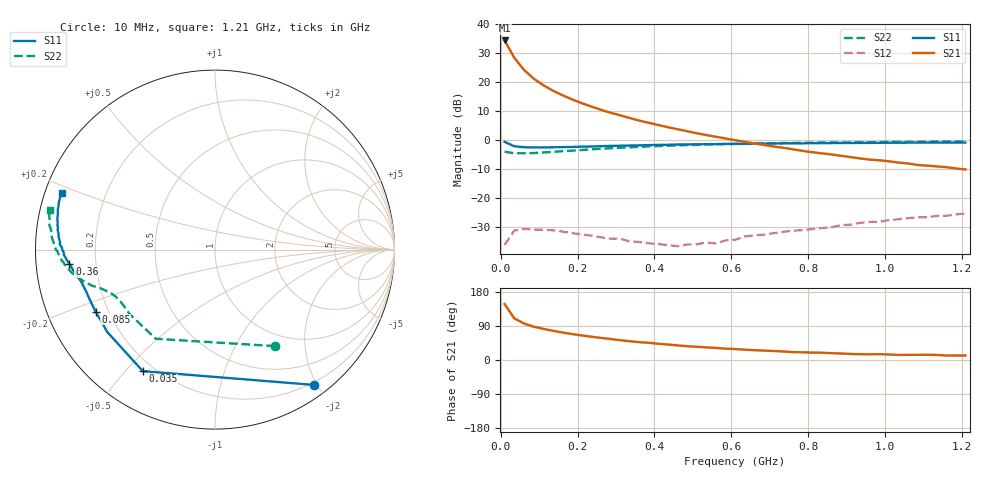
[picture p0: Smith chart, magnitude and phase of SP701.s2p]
!  POLYFET RF DEVICES
!  S PARAMETERS FOR
!  SP701
!  VDS=28, IDQ=200MA
! S1A1Die, AP pkg, Vds=28Vdc, Idq=200ma, Vgsth=2.60Vdc
! Date: Thu Jul 23 11:46:25 1998
# MHZ  S  MA  R  50.0000
! SCATTERING PARAMETERS :
! Freq=MHz Mag[s11] Ang[s11] Mag[s21] Ang[s21] Mag[s12] Ang[s12] Mag[s22] Ang[s22]
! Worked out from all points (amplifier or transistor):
!   49 points, 10 MHz to 1.21 GHz, reference 50 ohm
!   highest |S21| = 34.3 dB at 10 MHz (marker M1)
!   |S21| within 3 dB of that: start of sweep to 22.7 MHz
!   unconditionally stable (mu >= 1): 301.8 MHz to end of sweep
!   at 210 MHz: K = 0.66, MSG = 22.6 dB, |S12| = -32.4 dB
!   at 610 MHz: K = 1.67, MAG = 12.3 dB, |S12| = -34.3 dB
!   at 1.21 GHz: K = 1.05, MAG = 6.2 dB, |S12| = -25.2 dB
!   S11 on the Smith chart (normalised r, x): 10 MHz: 0.17, -1.96; 35 MHz: 0.16, -0.56; 85 MHz: 0.15, -0.24; 360 MHz: 0.10, -0.05; 1.21 GHz: 0.05, +0.18
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10  0.9341 -53.8  52.1 147.7  0.01566 58.0  0.6334 -58.1
35  0.7876 -120.7  26.4 110.0  0.02777 24.4  0.5962 -123.5
60  0.7556 -142.5  16.32 96.4  0.02968 13.1  0.5961 -142.8
85  0.7494 -152.6  11.58 88.1  0.02891 6.8  0.5998 -150.8
110  0.7513 -158.1  8.905 82.3  0.02883 3.8  0.6133 -154.9
135  0.754 -161.5  7.161 77.3  0.02807 -0.1  0.6291 -157.4
160  0.7599 -164.2  5.966 72.6  0.02676 1.2  0.6457 -159.0
185  0.7653 -166.3  5.057 68.6  0.02515 -1.8  0.6589 -160.2
210  0.7732 -167.7  4.357 65.0  0.0239 -2.3  0.6767 -161.6
235  0.7789 -169.2  3.81 61.5  0.02276 -1.1  0.6941 -162.6
260  0.7873 -170.5  3.349 58.4  0.02136 1.0  0.712 -163.5
285  0.7978 -171.5  2.981 55.5  0.02016 1.9  0.7265 -164.6
310  0.8024 -172.4  2.69 52.4  0.02029 5.4  0.7415 -165.5
360  0.8151 -174.4  2.177 47.1  0.01769 11.6  0.7672 -167.7
410  0.8289 -176.2  1.827 42.8  0.01626 20.8  0.7911 -169.8
485  0.8434 -178.9  1.427 36.4  0.01598 36.5  0.8241 -172.7
560  0.8558 178.9  1.146 31.8  0.01663 53.2  0.8472 -175.2
610  0.8634 177.5  1 28.9  0.01933 60.8  0.8633 -176.9
685  0.8756 175.0  0.8273 24.9  0.02369 68.3  0.8782 -179.5
810  0.8885 171.2  0.6223 19.6  0.02944 75.1  0.9038 176.8
1010  0.9037 165.6  0.4331 14.6  0.04196 82.2  0.9325 171.6
1210  0.9104 159.8  0.3131 11.9  0.05467 80.4  0.9447 166.7
